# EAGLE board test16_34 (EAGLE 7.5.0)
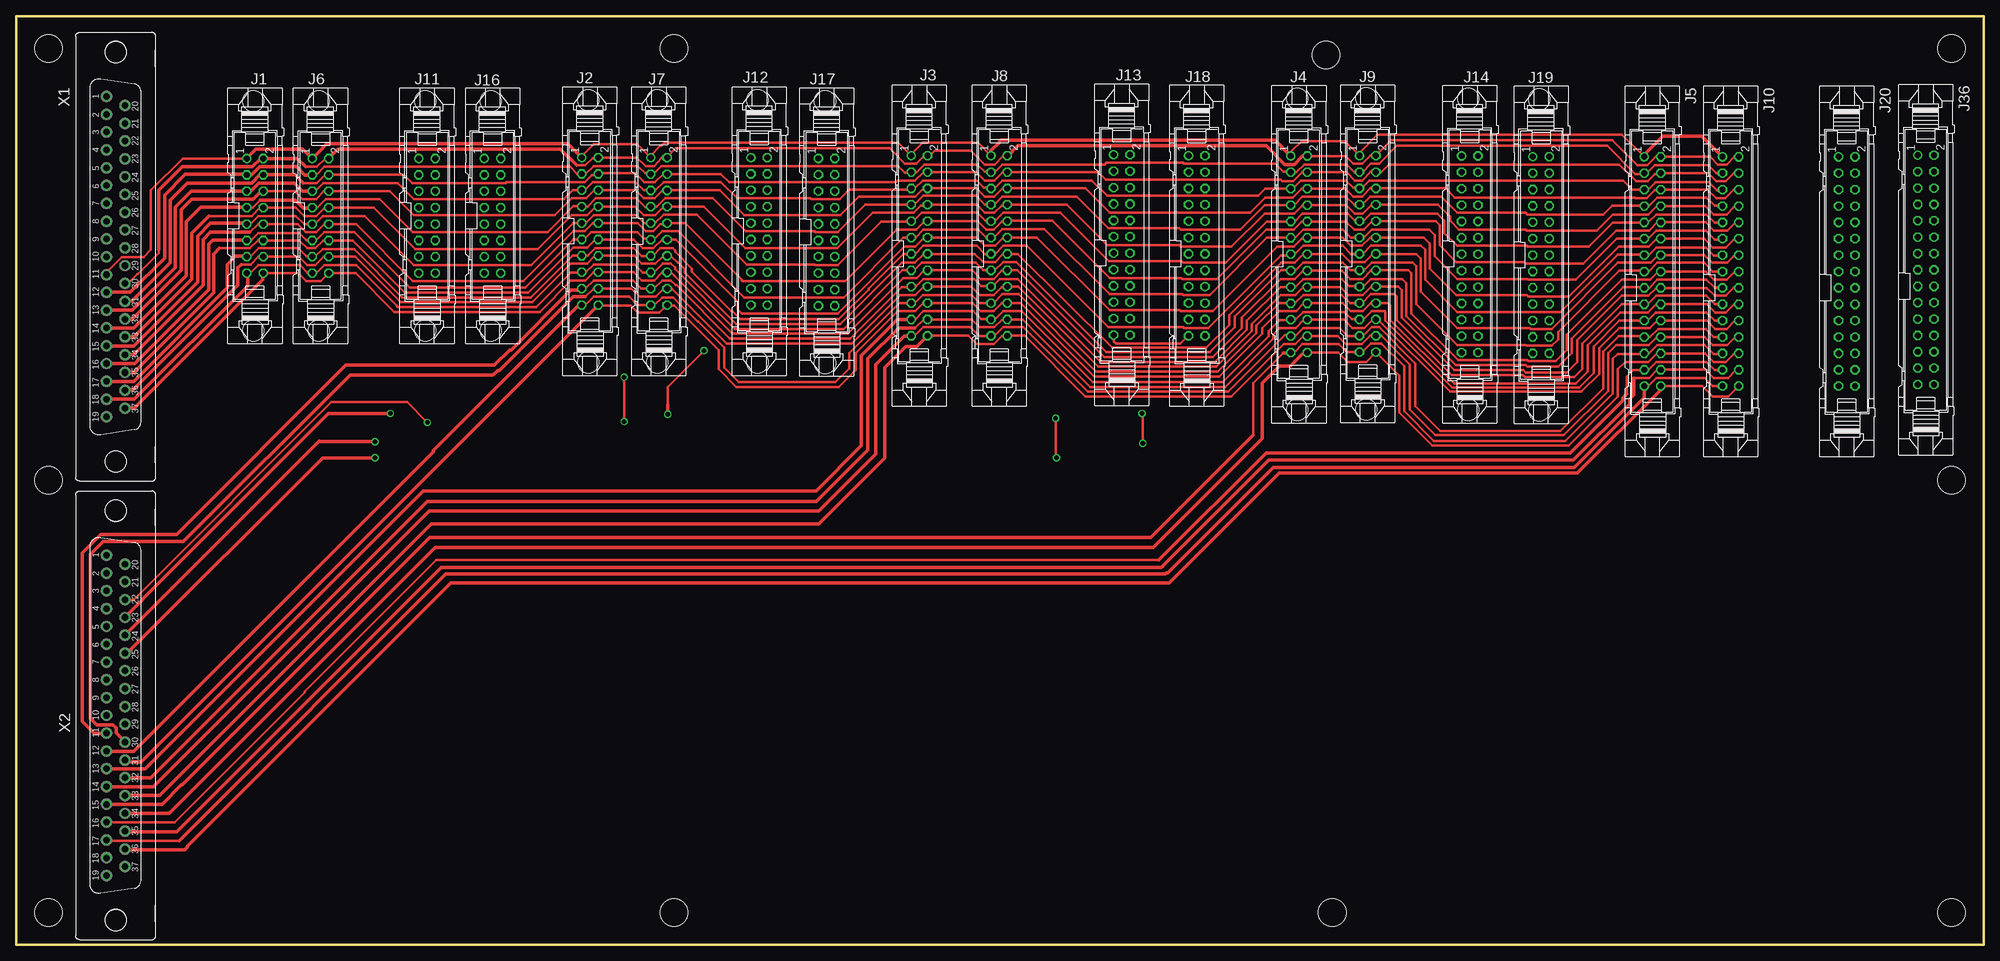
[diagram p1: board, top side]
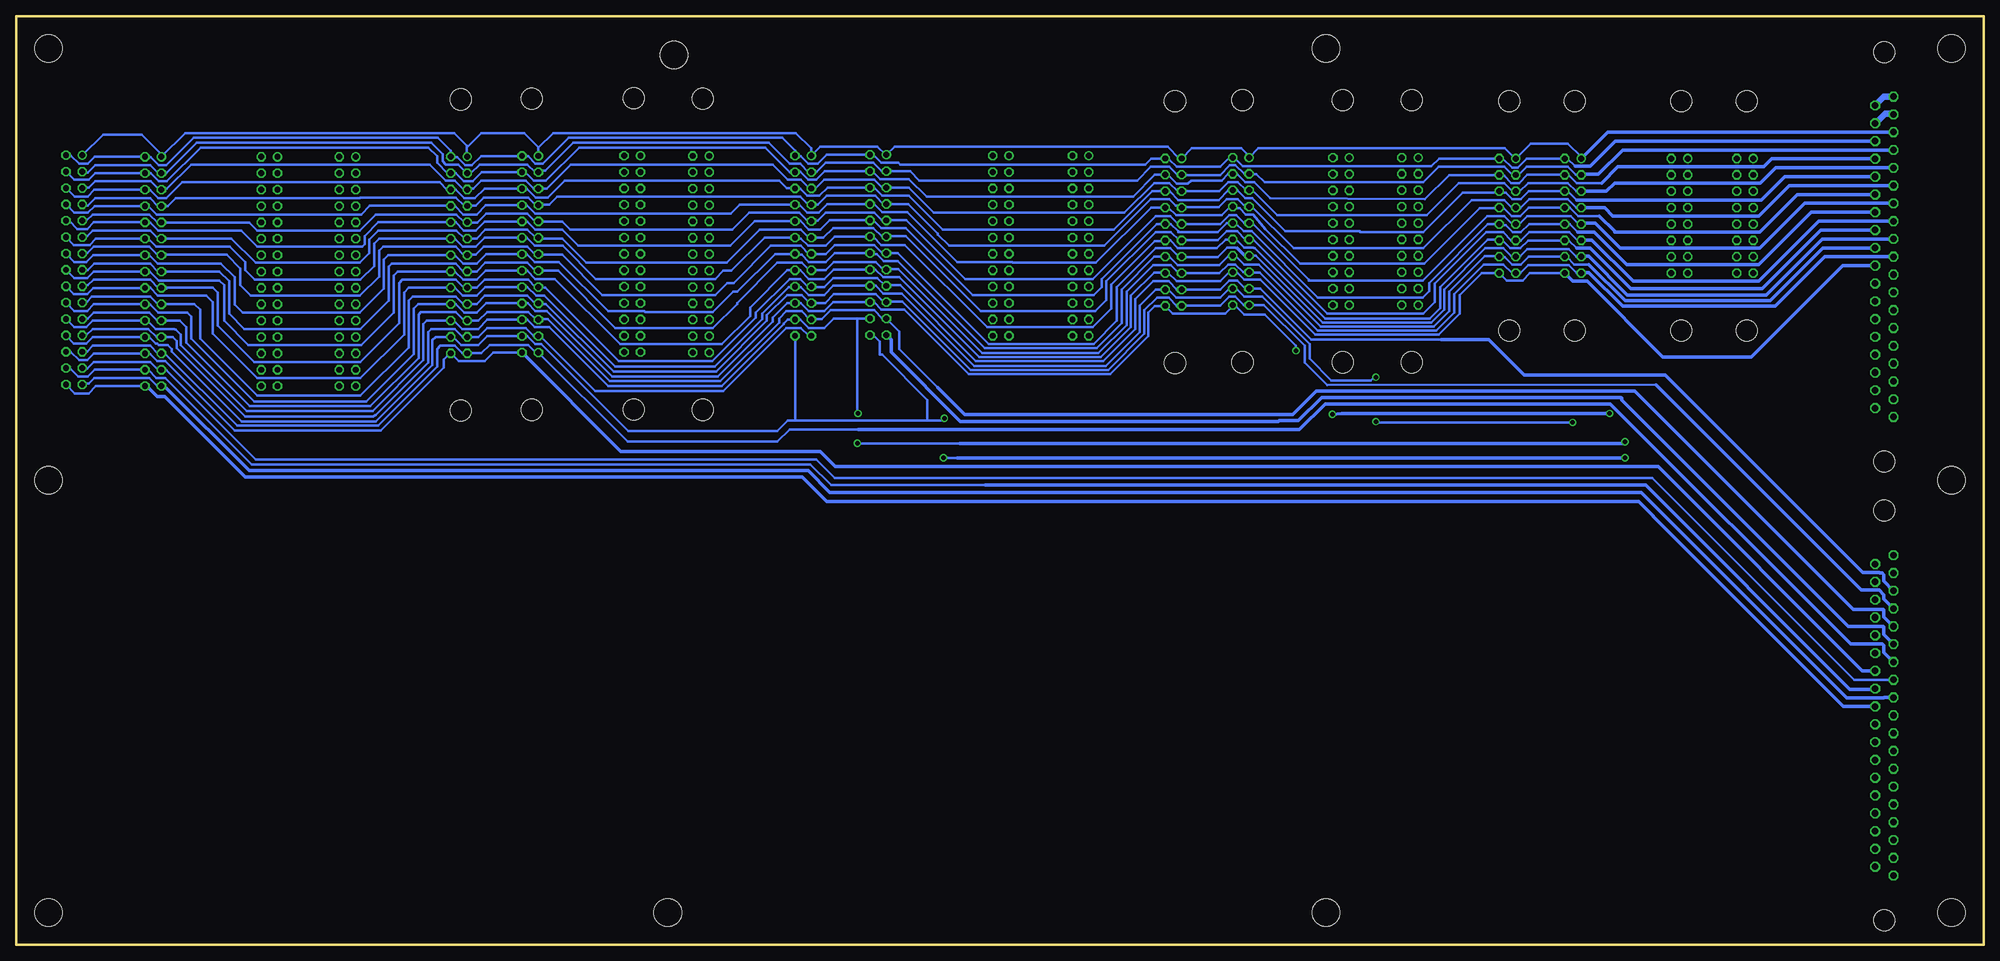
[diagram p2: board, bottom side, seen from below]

Size 305 x 144 mm. Coordinates in mm from the lower left corner, seen from the top.
Outline: 0,144 305,144 305,0 0,0 0,144
Copper layers (1*16): Top 0.035mm / dielectric 1.5mm / Bottom 0.035mm
Design rules "default": minimum track width 10mil, minimum drill 24mil, track to track 8mil, track to pad 8mil, pad to pad 8mil, via to via 8mil, smd to smd 8mil, copper to edge 40mil, drill to drill 8mil, minimum pad ring 10mil, minimum via ring 8mil, stop-mask expansion 4mil, vias tented up to drill 0mil, thermal gap 10mil
Holes 4.3 mm at 5,5 5,139 5,72 300,139 300,72 300,5 102,139 203,138 102,5 204,5

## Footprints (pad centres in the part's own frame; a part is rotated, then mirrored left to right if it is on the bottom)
16V = drill 0.914: 1 -8.89,-1.27 | drill 0.914 octagon: 2 -8.89,1.27; 3 -6.35,-1.27; 4 -6.35,1.27; 5 -3.81,-1.27; 6 -3.81,1.27; 7 -1.27,-1.27; 8 -1.27,1.27; 9 1.27,-1.27; 10 1.27,1.27; 11 3.81,-1.27; 12 3.81,1.27; 13 6.35,-1.27; 14 6.35,1.27; 15 8.89,-1.27; 16 8.89,1.27 | hole 3.302: 17.78,-0.254; -17.78,-0.254
20V = drill 0.914: 1 -11.43,-1.27 | drill 0.914 octagon: 2 -11.43,1.27; 3 -8.89,-1.27; 4 -8.89,1.27; 5 -6.35,-1.27; 6 -6.35,1.27; 7 -3.81,-1.27; 8 -3.81,1.27; 9 -1.27,-1.27; 10 -1.27,1.27; 11 1.27,-1.27; 12 1.27,1.27; 13 3.81,-1.27; 14 3.81,1.27; 15 6.35,-1.27; 16 6.35,1.27; 17 8.89,-1.27; 18 8.89,1.27; 19 11.43,-1.27; 20 11.43,1.27 | hole 3.302: 20.32,-0.254; -20.32,-0.254
24V = drill 0.914: 1 -15.24,-1.27 | drill 0.914 octagon: 2 -15.24,1.27; 3 -12.7,-1.27; 4 -12.7,1.27; 5 -10.16,-1.27; 6 -10.16,1.27; 7 -7.62,-1.27; 8 -7.62,1.27; 9 -5.08,-1.27; 10 -5.08,1.27; 11 -2.54,-1.27; 12 -2.54,1.27; 13 0,-1.27; 14 0,1.27; 15 2.54,-1.27; 16 2.54,1.27; 17 5.08,-1.27; 18 5.08,1.27; 19 7.62,-1.27; 20 7.62,1.27; 21 10.16,-1.27; 22 10.16,1.27; 23 12.7,-1.27; 24 12.7,1.27
26V = drill 0.914: 1 -15.24,-1.27 | drill 0.914 octagon: 2 -15.24,1.27; 3 -12.7,-1.27; 4 -12.7,1.27; 5 -10.16,-1.27; 6 -10.16,1.27; 7 -7.62,-1.27; 8 -7.62,1.27; 9 -5.08,-1.27; 10 -5.08,1.27; 11 -2.54,-1.27; 12 -2.54,1.27; 13 0,-1.27; 14 0,1.27; 15 2.54,-1.27; 16 2.54,1.27; 17 5.08,-1.27; 18 5.08,1.27; 19 7.62,-1.27; 20 7.62,1.27; 21 10.16,-1.27; 22 10.16,1.27; 23 12.7,-1.27; 24 12.7,1.27; 25 15.24,-1.27; 26 15.24,1.27 | hole 3.302: 24.13,-0.254; -24.13,-0.254
30V = drill 0.914: 1 -19.05,-1.27 | drill 0.914 octagon: 2 -19.05,1.27; 3 -16.51,-1.27; 4 -16.51,1.27; 5 -13.97,-1.27; 6 -13.97,1.27; 7 -11.43,-1.27; 8 -11.43,1.27; 9 -8.89,-1.27; 10 -8.89,1.27; 11 -6.35,-1.27; 12 -6.35,1.27; 13 -3.81,-1.27; 14 -3.81,1.27; 15 -1.27,-1.27; 16 -1.27,1.27; 17 1.27,-1.27; 18 1.27,1.27; 19 3.81,-1.27; 20 3.81,1.27; 21 6.35,-1.27; 22 6.35,1.27; 23 8.89,-1.27; 24 8.89,1.27; 25 11.43,-1.27; 26 11.43,1.27; 27 13.97,-1.27; 28 13.97,1.27; 29 16.51,-1.27; 30 16.51,1.27
F37V = drill 1.016 octagon: 1 24.841,1.422; 2 22.073,1.422; 3 19.329,1.422; 4 16.561,1.422; 5 13.792,1.422; 6 11.049,1.422; 7 8.28,1.422; 8 5.512,1.422; 9 2.769,1.422; 10 0,1.422; 11 -2.769,1.422; 12 -5.512,1.422; 13 -8.28,1.422; 14 -11.049,1.422; 15 -13.818,1.422; 16 -16.561,1.422; 17 -19.329,1.422; 18 -22.098,1.422; 19 -24.841,1.422; 20 23.47,-1.422; 21 20.701,-1.422; 22 17.932,-1.422; 23 15.189,-1.422; 24 12.421,-1.422; 25 9.652,-1.422; 26 6.909,-1.422; 27 4.14,-1.422; 28 1.372,-1.422; 29 -1.372,-1.422; 30 -4.14,-1.422; 31 -6.909,-1.422; 32 -9.677,-1.422; 33 -12.421,-1.422; 34 -15.189,-1.422; 35 -17.958,-1.422; 36 -20.701,-1.422; 37 -23.47,-1.422 | hole 3.302: 31.75,0; -31.75,0

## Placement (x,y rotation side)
J1  [16V]  37.02,113.03 270 top
J2  [20V]  88.94,110.64 270 top
J3  24VS  [24V]  140,107.12 270 top
J4  [26V]  198.84,107.08 270 top
J5  30V  [30V]  253.62,103.12 270 top
J6  [16V]  47.18,113.03 270 top
J7  [20V]  99.62,110.62 270 top
J8  24VS  [24V]  152.38,107.12 270 top
J9  [26V]  209.5,107.12 270 top
J10  30V  [30V]  265.75,103.12 270 top
J11  [16V]  63.69,113.03 270 top
J12  [20V]  115.17,110.64 270 top
J13  24VS  [24V]  171.38,107.25 270 top
J14  [26V]  225.31,107.08 270 top
J16  [16V]  73.85,113.03 270 top
J17  [20V]  125.62,110.5 270 top
J18  24VS  [24V]  183,107.12 270 top
J19  [26V]  236.37,106.95 270 top
J20  30V  [30V]  283.75,103.12 270 top
J36  30V  [30V]  296,103.38 270 top
X1  [F37V]  15.43,106.68 90 top
X2  [F37V]  15.43,35.56 90 top

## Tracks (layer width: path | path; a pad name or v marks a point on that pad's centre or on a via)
1
  Bottom 0.406: J11.1 62.42,122.17 64.5,124.25 70.25,124.25 J16.1 72.67,121.92 74.25,123.5 112.47,123.5 J12.1 113.89,122.27 115.12,123.5 122.78,123.5 J17.1 124.68,121.93 126.5,123.75 168.84,123.75 J13.1 170.24,122.49 171.5,123.75 180.34,123.75 J18.1 181.74,123.49 184.12,125.88 221.75,125.88 224.04,123.58 J14.1 224.04,123.67 226.25,125.88 232.88,125.88 235.12,123.62 | J19.1 235.12,122.22 235.12,123.62 | 235.12,123.62 235.12,123.88 237.12,125.88 278.78,125.88 J20.1 282.48,122.61 285.5,125.62 291.53,125.62 J36.1
  Bottom 0.506: X1.3 58.33,126.01 J11.1
2
  Bottom 0.406: 63.38,120.75 64.55,121.92 J11.2 70.83,121.92 72.25,120.5 73.12,120.5 74.55,121.92 J16.2 84.45,121.92 85.62,120.75 114.86,120.75 116.19,122.07 J12.2 116.93,122.07 118.38,120.62 125.12,120.62 126.25,121.75 126.72,121.75 J17.2 129.07,121.93 130,121 168,121 168.25,121.25 170.91,121.25 172.15,122.49 J13.2 179.38,122.49 180.75,121.12 182.25,121.12 183.38,122.25 184.16,122.25 J18.2 | 16.84,124.62 X1.22 | J18.2 184.27,122.52 | J18.2 184.27,123.14 186.25,125.12 219.38,125.12 223.38,121.12 224.5,121.12 225.62,122.25 226.51,122.25 J14.2 232.93,122.32 234.38,120.88 235.38,120.88 236.62,122.12 237.56,122.12 J19.2 237.63,123.14 239.62,125.12 277.5,125.12 281.75,120.88 282.88,120.88 284.12,122.12 284.97,122.12 J20.2 292.82,122.17 293.88,121.12 295.25,121.12 296.5,122.38 297.22,122.38 J36.2
  Bottom 0.506: X1.22 57.14,124.61 61,120.75 63.38,120.75
3
  Bottom 0.406: J11.3 63.26,119.38 64.5,120.62 70.88,120.62 72.12,119.38 J16.3 73.13,119.38 74.38,120.62 84.5,120.62 86.88,118.25 111.5,118.25 112.75,119.5 113.86,119.5 J12.3 114.66,119.53 116,120.88 116.88,120.88 118.38,119.38 124.34,119.38 J17.3 125.02,119.39 126.25,120.62 129.12,120.62 131.25,118.5 165,118.5 166.45,119.95 J13.3 170.82,119.95 172.12,121.25 179.5,121.25 180.88,119.88 181.68,119.88 J18.3 182.2,119.83 183.5,121.12 185.12,121.12 188.38,124.38 218.62,124.38 223,120 223.82,120 J14.3 224.53,119.78 225.75,121 233.12,121 234.5,119.62 235.06,119.62 J19.3 235.16,119.66 236.5,121 238.38,121 238.88,121.5 238.88,122.62 240.62,124.38 277,124.38 281.75,119.62 282.47,119.62 J20.3 283.01,119.64 284.25,120.88 292.75,120.88 293.88,119.75 294.6,119.75 J36.3 | 13.87,123.38 X1.4
  Bottom 0.506: X1.4 56.01,123.24 59.75,119.5 62.3,119.5 J11.3
4
  Bottom 0.406: 59.25,118.12 63.12,118.12 64.38,119.38 J11.4 70.75,119.38 72,118.12 73.25,118.12 74.38,119.25 74.99,119.25 J16.4 82.89,119.38 86.63,115.63 110.62,115.75 113.12,118.25 114.5,118.25 115.78,119.53 J12.4 117.09,119.53 118.12,118.5 122.88,118.5 123.38,118 125.13,118 126.52,119.39 J17.4 128.49,119.39 131.88,116 163.88,116 166.62,118.75 171.07,118.75 172.27,119.95 J13.4 179.68,119.95 181,118.62 182.25,118.62 183.5,119.88 184.22,119.88 J18.4 185.07,119.83 188.88,123.62 217.75,123.62 222.88,118.5 224.81,118.5 226.09,119.78 J14.4 232.84,119.78 234.25,118.38 235.62,118.38 236.88,119.62 237.6,119.62 J19.4 238.16,119.66 239.75,121.25 239.75,122.25 241.12,123.62 276.38,123.62 281.62,118.38 282.88,118.38 284.12,119.62 285.01,119.62 J20.4 286.49,119.64 286.5,119.62 292.75,119.62 293.75,118.62 296.01,118.62 J36.4 | X1.23
  Bottom 0.506: X1.23 32.88,121.87 34.12,120.62 56.75,120.62 59.25,118.12
5
  Bottom 0.406: J11.5 63.22,116.84 64.5,118.12 70.62,118.12 72,116.75 72.49,116.75 J16.5 73.09,116.84 74.38,118.12 81.38,118.12 86.38,113.12 109.5,113.12 113.36,116.99 J12.5 114.36,116.99 115.62,118.25 117.12,118.25 118.5,116.88 124.33,116.88 J17.5 124.97,116.85 126.25,118.12 128.62,118.12 133.25,113.5 162.75,113.5 166.66,117.41 J13.5 170.78,117.41 172,118.62 179.75,118.62 181.12,117.25 181.69,117.25 J18.5 182.03,117.28 183.38,118.62 185.38,118.62 187.75,121 219,121 222.75,117.25 J14.5 224.74,117.24 226,118.5 232.88,118.5 234.12,117.25 234.96,117.25 J19.5 235.62,117.11 237,118.5 238.38,118.5 240.88,121 277.88,121 281.62,117.25 282.32,117.25 J20.5 282.85,117.09 284.12,118.38 292.75,118.38 293.75,117.38 294.7,117.38 J36.5 | 13.98,120.5 X1.5
  Bottom 0.506: X1.5 32.28,120.47 34.62,118.12 57.25,118.12 58.5,116.88 62.38,116.88 J11.5
6
  Bottom 0.406: 63.12,115.5 64.47,116.84 J11.6 70.53,116.84 71.75,115.62 73.12,115.62 74.12,116.62 75,116.62 | 16.83,119.12 X1.24 | J16.6 75.12,116.75 75,116.62 | 75,116.62 80.75,116.62 86.88,110.5 96.62,110.5 96.75,110.62 108.25,110.62 113.38,115.75 114.5,115.75 115.74,116.99 J12.6 117.14,116.99 118.62,115.5 124.88,115.5 126.22,116.85 J17.6 128.9,116.85 134.88,110.88 161.38,110.88 166.62,116.12 170.74,116.12 172.02,117.41 J13.6 179.22,117.41 180.5,116.12 182.38,116.12 183.5,117.25 184.24,117.25 J18.6 185.53,117.28 186.75,118.5 220,118.5 222.62,115.88 224.47,115.88 225.84,117.24 J14.6 232.38,117.24 233.88,115.75 235.52,115.75 236.88,117.11 J19.6 238.24,117.11 239.38,118.25 279.25,118.25 281.75,115.75 283,115.75 284.25,117 284.93,117 J20.6 292.9,117.09 293.88,116 295.93,116 J36.6
  Bottom 0.506: X1.24 30.9,119.1 34.5,115.5 63.12,115.5
7
  Bottom 0.406: J11.7 63.17,114.3 64.5,115.62 70.5,115.62 71.88,114.25 72.53,114.25 J16.7 73.17,114.3 74.38,115.5 79.38,115.5 86.88,108 107,108 113.45,114.45 J12.7 114.45,114.45 115.62,115.62 117.38,115.62 118.62,114.38 124.29,114.38 J17.7 124.67,114.62 125.25,114.62 126.25,115.62 129.12,115.62 136.38,108.38 160.38,108.38 162.12,110.12 162.12,110.25 166.75,114.87 J13.7 170.62,114.87 171.88,116.12 179.38,116.12 180.75,114.75 J18.7 182.25,114.75 183.5,116 221.12,116 222.38,114.75 224,114.75 J14.7 224.45,114.7 225.62,115.88 232.5,115.88 233.75,114.62 235.04,114.62 J19.7 235.57,114.58 236.88,115.88 251.62,115.88 251.75,115.75 280.25,115.75 281.5,114.5 282.43,114.5 J20.7 283.06,114.56 284.25,115.75 292.75,115.75 293.88,114.62 294.55,114.62 J36.7 | 13.9,117.62 X1.6
  Bottom 0.506: X1.6 30.15,117.73 34.88,113 57.5,113 58.8,114.3 J11.7
8
  Bottom 0.406: 59.62,113 62.88,113 64.17,114.3 J11.8 70.58,114.3 71.88,113 73.19,113 74.5,114.3 J16.8 75.17,114.25 78.12,114.25 86.75,105.62 106,105.62 111.38,111 113.25,113.25 114.38,113.25 115.38,114.25 116.37,114.25 116.44,114.19 J12.8 116.8,114.45 118.12,113.12 125.21,113.12 126.39,114.31 J17.8 129.06,114.31 137.62,105.75 150.5,105.75 150.62,105.88 159.12,105.88 166.88,113.62 170.75,113.62 172,114.87 J13.8 179.25,114.87 180.62,113.5 182.4,113.5 183.65,114.75 J18.8 192.88,114.75 194.25,113.38 224.51,113.38 225.84,114.7 J14.8 232.18,114.7 233.62,113.25 235.69,113.25 237.01,114.58 J19.8 250.18,114.58 251.5,113.25 283.21,113.25 284.52,114.56 J20.8 292.82,114.56 293.88,113.5 295.96,113.5 J36.8 | 17.29,116.25 17.38,116.33
  Bottom 0.506: X1.25 17.38,116.33 28.92,116.33 34.75,110.5 57.25,110.5 57.25,110.62 59.62,113
9
  Bottom 0.406: J11.9 62.76,111.76 64,113 70.75,113 72,111.75 J16.9 73.14,111.76 74.38,113 77,113 87,103 104.61,103 104.61,103.11 113.25,111.75 113.73,111.75 J12.9 113.93,111.88 114.62,111.88 115.88,113.12 117,113.12 118.36,111.77 J17.9 124.89,111.77 126.12,113 128.38,113 138.12,103.25 157.88,103.25 167,112.38 170.06,112.38 J13.9 170.83,112.33 172,113.5 179.5,113.5 180.75,112.25 181.69,112.25 J18.9 182.33,112.2 183.62,113.5 191.38,113.5 194,110.88 219.12,110.88 220.38,112.12 224.01,112.12 J14.9 224.53,112.16 225.75,113.38 232.12,113.38 233.5,112 235.06,112 J19.9 235.53,112.03 236.75,113.25 249.25,113.25 251.75,110.75 267.62,110.75 268.88,112 282.46,112 J20.9 283.14,112.02 284.38,113.25 293.12,113.25 294.12,112.25 294.71,112.25 J36.9 | 13.97,115 X1.7
  Bottom 0.506: X1.7 27.79,114.96 34.75,108 56.38,108 60.25,111.88 62.3,111.88 J11.9
10
  Bottom 0.406: 16.82,113.62 X1.26 | 62.95,110.5 64.21,111.76 J11.10 70.49,111.76 71.75,110.5 73,110.5 74.12,111.62 74.98,111.62 J16.10 76.86,111.76 86,102.62 86,101.38 87,100.38 103.25,100.38 113.5,110.62 114.75,110.62 116.03,111.91 J12.10 117.34,111.91 118.75,110.5 124.88,110.5 124.88,110.62 126,111.75 126.88,111.75 J17.10 128.23,111.77 136.75,103.25 136.75,102 138,100.75 156.75,100.75 167.12,111.12 170.94,111.12 172.15,112.33 J13.10 178.92,112.33 180.38,110.88 182.12,110.88 183.5,112.25 184.22,112.25 J18.10 190.5,112.2 194.33,108.38 217.88,108.38 220.38,110.88 224.5,110.88 225.75,112.12 226.55,112.12 J14.10 232.34,112.16 233.75,110.75 235.6,110.75 236.88,112.03 J19.10 248.84,112.03 251,109.88 251,108.62 251.38,108.25 267.62,108.25 270.12,110.75 283,110.75 284.25,112 285,112 J20.10 292.99,112.02 294,111 295.5,111 296.75,112.25 297.25,112.25 J36.10
  Bottom 0.506: X1.26 26.79,113.59 34.88,105.5 55.38,105.5 60.38,110.5 62.95,110.5
11
  Bottom 0.406: 13.95,112.25 X1.8 | J11.11 62.97,109.22 64.25,110.5 70.5,110.5 71.78,109.22 J16.11 73.22,109.22 74.5,110.5 77.12,110.5 85.12,102.5 85.12,99.62 86.88,97.88 101.75,97.88 113.25,109.38 J12.11 114.5,109.37 115.75,110.62 117.38,110.62 118.77,109.23 J17.11 124.73,109.23 126,110.5 128.38,110.5 136,102.88 136,100 137.75,98.25 155.5,98.25 167.12,109.88 170.02,109.88 J13.11 170.79,109.79 172.12,111.12 178.38,111.12 179.88,109.62 181.69,109.62 J18.11 182.16,109.67 183.38,110.88 189.75,110.88 194.88,105.75 216.62,105.75 220.38,109.5 223.93,109.5 J14.11 224.5,109.62 225.75,110.88 232.25,110.88 233.62,109.5 J19.11 235.5,109.5 236.75,110.75 248.88,110.75 250.25,109.38 250.25,107.25 251.75,105.75 267.88,105.75 271.62,109.5 282.45,109.5 J20.11 282.98,109.47 284.25,110.75 293.12,110.75 294,109.88 294.58,109.88 J36.11
  Bottom 0.506: X1.8 25.56,112.19 34.88,102.88 54.38,102.88 60.75,109.25 62.39,109.25 J11.11
12
  Bottom 0.406: 63.12,108 64.34,109.22 J11.12 70.66,109.22 71.88,108 73.38,108 74.62,109.25 75.09,109.25 J16.12 75.28,109.38 76.88,109.38 84.25,102 84.25,98.75 85.88,97.12 102.12,97.12 113,108 113.12,108 113.25,108.12 114.62,108.12 115.87,109.37 J12.12 117.5,109.37 118.88,108 124.92,108 126.14,109.23 J17.12 127,109.12 128.5,109.12 135.25,102.38 135.25,98.62 138.12,95.75 154.5,95.75 167.25,108.5 170.88,108.5 172.16,109.79 J13.12 178.09,109.79 179.5,108.38 182.25,108.38 183.38,109.5 184.1,109.5 J18.12 189,109.67 194.16,104.5 195.38,104.5 196.62,103.25 215.12,103.25 220.25,108.38 224.59,108.38 225.84,109.62 J14.12 232.38,109.62 233.75,108.25 235.76,108.25 237.01,109.5 J19.12 248.75,109.5 249.5,108.75 249.5,105.25 251.62,103.12 268,103.12 269.5,104.62 269.5,105.88 271.88,108.25 283.3,108.25 284.52,109.47 J20.12 292.65,109.47 293.62,108.5 296.05,108.5 J36.12 | 16.8,110.88 X1.27
  Bottom 0.506: X1.27 25.3,110.82 34.38,101.75 54.75,101.75 61,108 63.12,108
13
  Bottom 0.406: J11.13 63.18,106.68 64.38,107.88 70.75,107.88 71.88,106.75 72.51,106.75 J16.13 72.65,106.75 73.25,106.75 74.5,108 77.25,108 83.62,101.62 83.62,98.5 85.62,96.5 102.5,96.5 112.83,106.83 J12.13 | 13.96,109.5 X1.9 | 115.75,108 115.88,108 116,108.12 117.25,108.12 118.75,106.62 124.29,106.62 J17.13 124.81,106.69 126.12,108 128.38,108 134.38,102 134.38,96.75 138,93.12 154.25,93.12 168.38,107.25 J13.13 170.75,107.25 172,108.5 178.12,108.5 179.5,107.12 J18.13 182.12,107.12 183.38,108.38 188,108.38 193.75,102.62 194.75,102.62 196.62,100.75 214.12,100.75 220.38,107 223.97,107 J14.13 | 223.84,106.88 J14.13 | J14.13 224.58,107.08 225.75,108.25 232.5,108.25 233.75,107 235.05,107 J19.13 235.58,106.95 236.88,108.25 248.12,108.25 248.75,107.62 248.75,103.62 251.75,100.62 268.62,100.62 270.25,102.25 270.25,104.88 272.38,107 282.42,107 J20.13 283.06,106.94 284.38,108.25 293,108.25 294,107.25 294.67,107.25 J36.13
  Bottom 0.506: X1.9 25.05,109.45 33.75,100.75 55.25,100.75 61.25,106.75 62.35,106.75 J11.13 | J12.13 114.58,106.83 115.75,108
14
  Bottom 0.406: 61.25,105.5 63.5,105.5 64.68,106.68 J11.14 70.57,106.68 71.75,105.5 73.12,105.5 74.25,106.62 75.06,106.62 J16.14 75.19,106.75 77.38,106.75 82.88,101.25 82.88,98.25 85.25,95.88 102.75,95.88 112.38,105.5 114.62,105.5 115.94,106.81 116.44,106.81 J12.14 117.05,106.83 118.5,105.38 124.95,105.38 126.27,106.69 J17.14 128.56,106.69 133.62,101.62 133.62,96.38 137.5,92.5 154.88,92.5 168.38,106 170.5,106 171.62,107.12 172.52,107.12 J13.14 178.12,107.25 179.5,105.88 182.12,105.88 183.25,107 184.15,107 J18.14 187.38,107.12 193.25,101.25 193.88,101.25 197,98.12 207.5,98.12 207.62,98.25 213.25,98.25 220.88,105.88 224.63,105.88 225.84,107.08 J14.14 232.17,107.08 233.62,105.62 235.68,105.62 237.01,106.95 J19.14 247.29,106.95 248,106.25 248,101.75 251.75,98 269.88,98 271.12,99.25 271.12,103.5 273.25,105.62 283.08,105.62 284.39,106.94 J20.14 293.06,106.94 294.12,105.88 295.96,105.88 J36.14 | 16.78,108.12 X1.28
  Bottom 0.506: X1.28 24.95,108.05 33.12,99.88 55.62,99.88 61.25,105.5
15
  Bottom 0.406: J11.15 63.14,104.14 64.38,105.38 70.62,105.38 71.88,104.12 72.56,104.12 J16.15 73.14,104.14 74.5,105.5 77.5,105.5 82.12,100.88 82.12,98 84.88,95.25 103.25,95.25 112.25,104.25 113.86,104.25 J12.15 114.79,104.29 116,105.5 117.12,105.5 118.5,104.12 124.33,104.12 J17.15 124.78,104.15 126,105.38 128.75,105.38 132.88,101.25 132.88,96.12 137.25,91.75 155.25,91.75 168.25,104.75 170.06,104.75 J13.15 170.59,104.71 171.75,105.88 178.25,105.88 179.5,104.62 181.69,104.62 J18.15 182.09,104.58 183.25,105.75 187,105.75 193.25,99.5 193.25,99.38 197,95.62 212.12,95.62 221,104.5 224,104.5 J14.15 224.54,104.54 225.75,105.75 232.25,105.75 233.62,104.38 235.06,104.38 J19.15 235.66,104.42 236.88,105.62 246.75,105.62 247.25,105.12 247.25,99.88 251.62,95.5 269.62,95.5 272,97.88 272,102.88 273.5,104.38 282.46,104.38 J20.15 283.02,104.39 284.25,105.62 292.88,105.62 293.88,104.62 294.71,104.62 J36.15 | 13.95,106.62 X1.10
  Bottom 0.506: X1.10 24.7,106.68 32.38,99 56,99 61.25,104.25 62.31,104.25 J11.15
16
  Bottom 0.406: J11.16 70.36,104.14 71.5,103 73.98,103 J16.16 77.86,104.14 81.25,100.75 81.25,97.88 84.5,94.62 103.62,94.62 112.12,103.12 114.62,103.12 115.79,104.29 J12.16 116.96,104.29 118.38,102.88 125.12,102.88 126.39,104.15 J17.16 127,104.25 128.62,104.25 132.25,100.62 132.25,95.75 136.88,91.12 155.75,91.12 168.12,103.5 170.62,103.5 171.84,104.71 J13.16 178.29,104.71 179.75,103.25 182.12,103.25 183.5,104.62 184.23,104.62 J18.16 185.5,104.58 191.25,98.83 191.25,97.5 195.62,93.12 211.38,93.12 221.5,103.25 224.5,103.25 225.75,104.5 226.54,104.5 J14.16 232.21,104.54 233.62,103.12 235.72,103.12 237.01,104.42 J19.16 245.84,104.42 246.5,103.75 246.5,98 251.5,93 269,93 272.75,96.75 272.75,102.25 273.5,103 282.88,103 284.27,104.39 J20.16 292.98,104.39 294,103.38 296,103.38 J36.16 | 16.79,105.25 X1.29
  Bottom 0.506: X1.29 21.88,105.31 36.06,91.12 49.75,91.12 61.5,102.88 63.7,102.88 J11.16
17
  Bottom 0.406: 84.12,93.88 104.25,93.88 112.12,101.75 J12.17 114.5,101.75 115.75,103 117,103 118.38,101.62 124.34,101.62 J17.17 125.11,101.61 126.38,102.88 128.75,102.88 131.5,100.12 131.5,95.5 136.5,90.5 156.25,90.5 168,102.25 170.03,102.25 J13.17 170.29,102.17 171.5,103.38 178.38,103.38 179.75,102 181.69,102 J18.17 182.29,102.05 183.5,103.25 185.12,103.25 190.38,98 190.38,97.25 197.12,90.5 211.62,90.5 223,101.88 223.92,101.88 J14.17 224.5,102 225.62,103.12 232.38,103.12 233.62,101.88 J19.17 235.62,101.88 236.88,103.12 245.12,103.12 245.62,102.62 245.62,96.38 251.62,90.38 268.12,90.38 273.75,96 273.75,101.12 274.5,101.88 281.62,101.88 281.75,101.75 282.38,101.75 J20.17 282.98,101.86 284.25,103.12 293,103.12 293.88,102.25 294.58,102.25 J36.17
  Bottom 0.506: X2.3 15.5,56.38 15.5,57.38 15.75,57.62 16.12,57.62 16.25,57.75 18.75,57.75 49.38,88.38 71.25,88.38 76.75,93.88 84.12,93.88
18  (via drill 0.7)
  Top 0.406: X2.22 18.24,53.49 48.88,84.12 60.62,84.12 v63.75,81 | v94.25,81.12 v94.25,88
  Bottom 0.406: v63.75,81 94.12,81 v94.25,81.12 | 116.44,101.69 115.81,101.69 114.62,100.5 111.88,100.5 104.5,93.12 104.5,90.88 101.12,87.5 95,87.5 94.5,88 v94.25,88 | 116.44,101.69 117.06,101.69 118.38,100.38 125.16,100.38 126.39,101.61 J17.18 126.91,101.62 128.38,101.62 130.88,99.12 130.88,95 136.12,89.75 156.5,89.75 167.75,101 170.62,101 171.79,102.17 J13.18 178.33,102.17 179.75,100.75 182.12,100.75 183.38,102 184.22,102 J18.18 184.31,102 185.25,102 189.38,97.88 189.38,97 196.75,89.62 212.12,89.62 223.12,100.62 224.38,100.62 225.75,102 J14.18 232.25,102 233.62,100.62 235.76,100.62 237.01,101.88 J19.18 244.12,101.88 244.88,101.12 244.88,94.62 251.62,87.88 267.62,87.88 274.5,94.75 274.5,99.62 275.5,100.62 283.04,100.62 283.04,100.67 284.25,101.88 285,101.88 J20.18 293.02,101.86 294,100.88 296.04,100.88 J36.18
  Bottom 0.506: 116.44,101.69 J12.18
19
  Bottom 0.406: 50.81,86.81 50.88,86.88 101.75,86.75 105.25,90.25 105.25,92.88 111.58,99.21 J12.19 114.71,99.21 116,100.5 117,100.5 118.38,99.12 124.3,99.12 J17.19 125.07,99.07 126.38,100.38 128.12,100.38 130.12,98.38 130.12,94.75 135.75,89.12 157,89.12 167.62,99.75 169.99,99.75 J13.19 170.5,99.63 171.75,100.88 178.25,100.88 179.62,99.5 J18.19 182,99.5 183.25,100.75 185.5,100.75 188.62,97.62 188.62,96.75 196.5,88.88 212.38,88.88 222.88,99.38 223.96,99.38 J14.19 | 224,99.5 J14.19 | J14.19 224.59,99.46 225.75,100.62 232.38,100.62 233.62,99.38 235.06,99.38 J19.19 235.71,99.33 236.88,100.5 243.5,100.5 244.12,99.88 244.12,92.62 251.62,85.12 267.62,85.12 276.5,94 276.5,98.5 277.38,99.38 282.42,99.38 J20.19 283.06,99.31 284.25,100.5 293.25,100.5 294,99.75 294.55,99.75 J36.19
  Bottom 0.506: X2.4 15.5,53.61 15.5,54.25 16.25,55 19,55 50.81,86.81
20  (via drill 0.7)
  Top 0.406: 101,83.78 101,86.5 v106.62,92.12
  Top 0.506: X2.23 19.62,53.52 19.62,53.62 48.38,82.38 v58,82.38 | v101,82.25 101,83.78
  Bottom 0.406: v106.62,92.12 106.62,92.88 111.5,97.75 114.62,97.75 116.08,99.21 J12.20 116.44,99.06 117.62,97.88 125.7,97.88 J17.20 126.97,99 128.5,99 129.5,98 129.5,94.38 135.38,88.5 157.38,88.5 167.38,98.5 170.88,98.5 172,99.63 J13.20 178.37,99.63 179.75,98.25 182.12,98.25 183.38,99.5 J18.20 185.5,99.5 187.75,97.25 187.75,96.62 196.25,88.12 212.62,88.12 222.75,98.25 224.5,98.25 225.71,99.46 J14.20 232.16,99.46 233.62,98 235.55,98 236.88,99.33 J19.20 242.66,99.33 243.38,98.62 243.38,91.62 250.75,84.25 268.12,84.25 277.88,94 277.88,97.38 278.5,98 283,98 284.25,99.25 284.95,99.25 J20.20 292.94,99.31 294,98.25 295.95,98.25 J36.20
  Bottom 0.506: v58,82.38 99.5,82.38 v101,82.25
21
  Bottom 0.406: 162.12,86.38 168.12,92.38 168.12,95.11 J13.21 170.72,97.09 172,98.38 178.75,98.38 180.12,97 181.69,97 J18.21 181.97,96.97 183.25,98.25 185.62,98.25 186.75,97.12 186.75,96.5 195.88,87.38 213,87.38 222.62,97 223.97,97 J14.21 224.42,96.92 225.62,98.12 232,98.12 233.38,96.75 235.05,96.75 J19.21 235.54,96.8 236.88,98.12 242.25,98.12 242.62,97.75 242.62,91 250.12,83.5 268.75,83.5 278.62,93.38 278.62,95.75 279.62,96.75 282.45,96.75 J20.21 283.15,96.78 284.38,98 293,98 293.88,97.12 294.63,97.12 J36.21
  Bottom 0.506: X2.5 15.5,50.84 15.5,51.88 15.62,52 20.25,52 54.12,85.88 103.5,85.88 107.12,82.25 158,82.25 162.12,86.38
22  (via drill 0.7)
  Top 0.406: v174.62,77.75 174.62,82.25 v174.5,82.38
  Top 0.506: X2.24 46.87,78 | 46.87,78 47,78.12 | v55.62,78 46.87,78
  Bottom 0.406: 172.78,97.09 J13.22 172.68,97.12 174.5,97.12 | 174.62,82.75 174.62,97 174.5,97.12 | 174.62,82.75 174.62,82.5 v174.5,82.38 | v174.5,82.38 174.38,82.25 | 158.75,77.75 v174.62,77.75 | v174.5,82.38 174.5,82.62 174.62,82.75 | 174.5,97.12 178.25,97.12 179.75,95.62 182.12,95.62 183.47,96.97 J18.22 185.38,96.97 186,96.34 186,96.25 195.62,86.62 213.25,86.62 222.38,95.75 224.62,95.75 225.79,96.92 J14.22 231.96,96.92 233.38,95.5 235.84,95.5 237.13,96.8 J19.22 241.33,96.8 241.88,96.25 241.88,90.62 249.75,82.75 269.25,82.75 279.5,93 279.5,94.62 280.25,95.38 280.38,95.38 280.5,95.5 283.38,95.5 284.65,96.78 J20.22 293.1,96.78 294.12,95.75 296,95.75 J36.22
  Bottom 0.506: 158.75,77.75 55.88,77.75 v55.62,78
23
  Top 0.406: J18.23 180.43,93.25 170.5,93.25 170.1,93.52 J13.23
  Bottom 0.406: J18.23 182.18,94.42 183.38,95.62 185.62,95.62 195.38,85.88 215.25,85.88 223.5,94.12 223.79,94.12 J14.23 224.75,94.38 226,95.62 232,95.62 233.38,94.25 J19.23 235.75,94.25 237,95.5 240.62,95.5 241.12,95 241.12,90.25 249.25,82.12 249.38,82.12 249.62,81.88 269.5,81.88 280.12,92.5 280.12,93.62 280.75,94.25 282.46,94.25 J20.23 283.24,94.23 284.5,95.5 293.12,95.5 294.12,94.5 294.71,94.5 J36.23
  Bottom 0.506: X2.6 15.5,48.1 15.5,49.25 15.62,49.38 21,49.38 56.12,84.5 56.12,84.75 56.25,84.88 102.62,84.88 106.25,81.25 109.25,81.25 109.38,81.12 158.62,81.12 169.38,91.88 169.38,93.82 J13.23
24  (via drill 0.7)
  Top 0.406: v161.12,81.62 161.12,75.62 v161.25,75.5
  Top 0.506: v55.62,75.5 47.5,75.5 17.38,45.38 17.02,45.38 X2.25
  Bottom 0.406: v161.25,75.5 159.12,75.5 | J18.24 184.27,81.48 184.5,81.25 | 184.5,81.25 163.88,81.25 | 163.88,81.25 161.5,81.25 v161.12,81.62 | 163.88,81.25 163.75,81.38 163.75,84.5 170.75,91.5 171.12,91.5 171.12,93.5 172.15,94.52 172.62,94.52 J13.24 | 184.5,81.25 185.38,81.25 187,79.62 210.12,79.62 223.62,93.12 224.5,93.12 225.75,94.38 225.88,94.38 J14.24 232,94.38 233.38,93 236,93 237.26,94.25 J19.24 240,94.25 240.5,93.75 240.5,89.88 249.25,81.12 270,81.12 280.88,92 280.88,92.38 281.5,93 282.91,93 283.16,93.25 283.38,93.25 284.36,94.23 J20.24 293.14,94.23 294.12,93.25 296.04,93.25 J36.24
  Bottom 0.506: 159.12,75.5 v55.62,75.5
25
  Bottom 0.406: 174.5,79.88 185.12,79.88 187,78 210.21,78 J14.25 224.47,91.84 225.62,93 231.62,93 232.88,91.75 235.06,91.75 J19.25 235.84,91.72 237,92.88 239.25,92.88 239.75,92.38 239.75,89.62 248.88,80.5 270.75,80.5 281.88,91.62 282.41,91.62 J20.25 283.07,91.69 284.25,92.88 293.12,92.88 294,92 294.68,92 J36.25
  Bottom 0.506: X2.7 15.5,45.33 15.5,46.38 15.75,46.62 20.62,46.62 57.88,83.88 102.12,83.88 106.12,79.88 174.5,79.88
26
  Bottom 0.406: J14.26 231.03,91.84 232.38,90.5 236.42,90.5 J19.26 237.78,91.72 238.75,90.75 238.75,89.5 248.5,79.75 271.12,79.75 281.88,90.5 283.12,90.5 284.25,91.62 284.95,91.62 J20.26 292.93,91.69 294,90.62 295.25,90.62 296.5,91.88 297.2,91.88 J36.26
  Bottom 0.506: X2.26 18.84,42.47 50.5,74.12 178,74.12 180.38,76.5 211.25,76.5 J14.26
27
  Bottom 0.406: X2.8 20.07,41.07 51.38,72.38 178.12,72.38 181,75.25 267.88,75.25 281.62,89 282.32,89 J20.27 283.03,89.16 284.25,90.38 293,90.38 294,89.38 294.7,89.38 J36.27
28
  Bottom 0.406: 154.75,71.25 178.62,71.25 181.88,74.5 268.5,74.5 281.88,87.88 283.25,87.88 284.53,89.16 J20.28 292.85,89.16 293.88,88.12 295.38,88.12 296.62,89.38 297.24,89.38 J36.28
  Bottom 0.506: 154.75,71.25 52.38,71.25 20.75,39.62 16.93,39.62 X2.27
29
  Bottom 0.406: J20.29 283.12,86.61 284.38,87.88 292.88,87.88 293.75,87 294.6,87 J36.29
  Bottom 0.506: X2.9 15.42,38.33 15.5,38.25 21.25,38.25 53.12,70.12 178.88,70.12 182.25,73.5 268.88,73.5 281.88,86.5 282.37,86.5 J20.29
30
  Bottom 0.406: J20.30 292.63,86.61 293.75,85.5 295.9,85.5 J36.30
  Bottom 0.506: J20.30 284.74,86.61 283.12,85 282,85 269.5,72.5 183.12,72.5 179.38,68.75 53.5,68.75 51.25,66.5 51.25,66.38 21.81,36.93 X2.28
+5V
  Bottom 1.016: X1.21 16.74,127.38 15.25,128.88 14.13,128.88 X1.2
GND
  Bottom 1.016: X1.1 15.48,131.52 X1.20
L1
  Top 0.406: J2.1 87.67,122.3 89.5,124.12 96.28,124.12 J7.1 98.36,122.36 99.88,123.88 100,123.88 100.5,124.38 136.72,124.38 J3.1 138.73,122.61 140.5,124.38 149.09,124.38 J8.1 | J1.1 25.8,121.92 20.88,117 20.88,107.75 19.75,106.62 16.38,106.62 14.38,104.62 14.38,104.28 X1.11 | J4.1 197.57,122.94 199.25,124.62 205.97,124.62 J9.1 208.23,122.86 211,125.62 248.91,125.62 J5.1
  Top 0.506: J1.1 35.75,122 37.12,123.38 44.45,123.38 J6.1 47.5,123.5 47.5,123.62 48.12,124.25 85.49,124.25 J2.1 | J8.1 151.1,123.11 152.38,124.38 152.38,124.5 152.62,124.75 195.14,124.75 J4.1 | J5.1 252.35,122.48 255.25,125.38 261.28,125.38 J10.1
L2
  Top 0.406: 86.88,120.88 88.25,120.88 89.38,122 90.14,122 J2.2 96.18,122.07 97.62,120.75 98.88,120.75 100.06,122.06 J7.2 100.89,122.14 102.25,123.5 135.38,123.5 137.75,121.12 139.53,121.12 140.77,122.36 J3.2 141.62,122.36 142.38,123.12 148,123.12 150.12,121 151.66,121 153.02,122.36 J8.2 | J6.2 47.92,121.92 46.62,120.62 44.88,120.62 | 22.12,107.75 22.12,107.25 18.88,104 18.75,104 17.38,102.62 16.94,102.62 X1.30 | J4.2 202.68,122.32 202.75,122.25 206.12,122.25 207.25,121.12 208.62,121.12 209.88,122.38 210.76,122.38 J9.2 210.77,122.39 213.12,124.75 247.38,124.75 251.25,120.88 252.84,120.88 254.15,122.17 J5.2 262.57,122.17 263.75,121 265.12,121 266.3,122.17 J10.2
  Top 0.506: 22.12,107.75 22.12,117 25.75,120.62 36.62,120.62 37.92,121.92 J1.2 43.58,121.92 44.88,120.62 | J6.2 48.45,121.95 49.88,123.38 84.38,123.38 86.88,120.88 | J8.2 153.74,122.36 155.25,123.88 193.75,123.88 196.62,121 198.12,121 199.38,122.25 200.04,122.25 J4.2
L3
  Top 0.406: J6.3 46.5,119.38 47.75,120.62 85.88,120.62 87,119.5 87.64,119.5 J2.3 88.28,119.53 89.5,120.75 96.38,120.75 97.5,119.62 98.25,119.62 J7.3 98.77,119.52 100,120.75 136.75,120.75 137.75,119.75 138.66,119.75 J3.3 139.57,119.83 140.75,121 149,121 150.12,119.88 151.06,119.88 J8.3 151.7,119.83 152.88,121 168.75,121 169,121.25 180.88,121.25 181,121.12 195.12,121.12 196.38,119.88 197.47,119.88 J4.3 198.41,119.78 199.62,121 206.25,121 207.5,119.75 208.16,119.75 J9.3 208.7,119.83 210,121.12 211.25,121.12 214,123.88 246.62,123.88 251,119.5 252.22,119.5 J5.3 252.76,119.64 254,120.88 262.25,120.88 263.5,119.62 264.47,119.62 J10.3
  Top 0.506: X1.12 17.67,101.17 23,106.5 23,116.25 26.25,119.5 35.63,119.5 J1.3 36.51,119.38 37.75,120.62 43.5,120.62 44.75,119.38 J6.3
L4
  Top 0.406: 44.5,118.12 46.62,118.12 47.88,119.38 J6.4 60.12,119.38 61.38,118.12 75.88,118.12 76,118.25 88.12,118.25 89.25,119.38 90.06,119.38 J2.4 90.31,119.62 96,119.62 97.38,118.25 99,118.25 100.27,119.52 J7.4 109.23,119.52 110.5,118.25 136.38,118.25 136.62,118.5 139.32,118.5 140.65,119.83 J3.4 148.8,119.83 150.12,118.5 151.62,118.5 152.88,119.75 153.57,119.75 J8.4 167.68,119.83 168.88,118.62 196,118.62 196.25,118.38 197.96,118.38 199.36,119.78 J4.4 206.22,119.78 207.5,118.5 208.62,118.5 210,119.88 210.72,119.88 J9.4 211.57,119.83 212.75,121 248.5,121 251.12,118.38 252.88,118.38 254,119.5 254.76,119.5 J5.4 262.24,119.64 263.5,118.38 265,118.38 266.25,119.62 267.01,119.62 J10.4
  Top 0.506: X1.31 17.9,99.77 23.88,105.75 23.88,115.5 26.5,118.12 36.5,118.12 37.76,119.38 J1.4 43.24,119.38 44.5,118.12
L5
  Top 0.406: J6.5 46.34,116.84 47.62,118.12 59.12,118.12 61.62,115.62 84.88,115.62 86.25,117 J2.5 88.11,116.99 89.38,118.25 96,118.25 97.25,117 98.33,117 J7.5 99.1,116.97 100.38,118.25 109.25,118.25 111.75,115.75 123.12,115.75 123.25,115.62 127.62,115.62 129.12,117.12 138.57,117.12 J3.5 139.28,117.28 140.5,118.5 148.88,118.5 150,117.38 151.01,117.38 J8.5 151.66,117.28 152.88,118.5 166.75,118.5 169.12,116.12 192.5,116.12 193.62,117.24 J4.5 197.87,117.24 199.12,118.5 206.12,118.5 207.25,117.38 208.14,117.38 J9.5 208.53,117.28 209.75,118.5 249.12,118.5 250.5,117.12 252.32,117.12 J5.5 252.97,117.09 254.12,118.25 262.38,118.25 263.62,117 264.38,117 J10.5
  Top 0.506: X1.13 18.02,98.4 24.62,105 24.62,114.38 27.12,116.88 35.72,116.88 J1.5 36.34,116.84 37.62,118.12 43.12,118.12 44.38,116.88 45.88,116.88 J6.5
L6
  Top 0.406: J1.6 43.16,116.84 44.38,115.62 46.5,115.62 47.72,116.84 J6.6 57.91,116.84 61.62,113.12 83.5,113.12 86.12,115.75 88.38,115.75 89.61,116.99 J2.6 96.01,116.99 97.25,115.75 99,115.75 100.22,116.97 J7.6 109.03,116.97 112.88,113.12 127.75,113.12 130.62,116 139.36,116 140.65,117.28 J3.6 148.84,117.28 150.12,116 151.62,116 152.88,117.25 153.61,117.25 J8.6 165.72,117.28 169.5,113.5 191.25,113.5 193.62,115.88 197.87,115.88 199.24,117.24 J4.6 206.01,117.24 207.25,116 208.61,116 209.9,117.28 J9.6 221.59,117.28 223,115.88 250.88,115.88 251,115.75 252.75,115.75 254,117 254.8,117 J5.6 262.15,117.09 263.5,115.75 264.88,115.75 266.25,117.12 266.99,117.12 J10.6
  Top 0.506: X1.32 18,97 25.62,104.62 25.62,114 27.25,115.62 36.75,115.62 37.97,116.84 J1.6
L7
  Top 0.406: 37.88,115.5 36.67,114.3 J1.7 | J6.7 46.67,114.3 48,115.62 56.38,115.62 61.5,110.5 82.38,110.5 86.38,114.5 87.62,114.5 J2.7 88.58,114.45 89.88,115.75 96.12,115.75 97.5,114.38 98.3,114.38 J7.7 99.31,114.44 100.62,115.75 108,115.75 113.12,110.62 123.75,110.62 123.88,110.5 127.38,110.5 131.62,114.75 J3.7 139.25,114.75 140.62,116.12 148.75,116.12 150.12,114.75 J8.7 151.62,114.75 152.88,116 164.38,116 169.25,111.12 180.25,111.12 180.5,110.88 189.75,110.88 193.57,114.7 J4.7 198.07,114.7 199.38,116 206.12,116 207.38,114.75 J9.7 208.62,114.75 209.88,116 220.88,116 223.38,113.5 234,113.5 234.25,113.25 246,113.25 247.38,114.62 252.28,114.62 J5.7 253.06,114.56 254.38,115.88 262,115.88 263.25,114.62 264.41,114.62 J10.7
  Top 0.506: X1.14 18.26,95.63 26.38,103.75 26.38,112.12 28.62,114.38 35.67,114.38 J1.7 | 37.88,115.5 43.25,115.5 44.5,114.25 45.86,114.25 J6.7
L8
  Top 0.406: 29.88,113 36.5,113 37.8,114.3 J1.8 43.33,114.3 44.62,113 46.5,113 47.8,114.3 J6.8 55.45,114.3 61.88,107.88 80.88,107.88 86.12,113.12 88.51,113.12 89.83,114.45 J2.8 95.92,114.45 97.25,113.12 99.08,113.12 100.39,114.44 J7.8 106.56,114.44 113,108 127.25,108 132.75,113.5 139.12,113.5 140.25,114.62 141.15,114.62 J3.8 148.88,114.75 150.12,113.5 151.62,113.5 152.75,114.62 153.53,114.62 J8.8 162.88,114.75 169.12,108.5 180.25,108.5 180.5,108.25 188.38,108.25 193.5,113.38 198.12,113.38 199.45,114.7 J4.8 206.18,114.7 207.5,113.38 208.75,113.38 210.12,114.75 J9.8 220.38,114.75 222.25,112.87 222.25,112.25 223.62,110.88 234,110.88 234.12,110.75 245,110.75 247.5,113.25 252.97,113.25 254.27,114.56 J5.8 261.82,114.56 263.12,113.25 265.12,113.25 266.25,114.38 266.84,114.38 J10.8
  Top 0.506: X1.33 18.26,94.26 27.25,103.25 27.25,110.38 29.88,113
L9
  Top 0.406: J1.9 36.26,111.76 37.5,113 43.38,113 44.62,111.75 J6.9 46.26,111.76 47.5,113 54,113 61.62,105.38 79.88,105.38 86.38,111.88 87.64,111.88 J2.9 88.28,111.91 89.5,113.12 96.12,113.12 97.38,111.88 98.33,111.88 J7.9 99.02,111.89 100.38,113.25 105.5,113.25 113.25,105.5 123.75,105.5 123.88,105.38 127.38,105.38 134.12,112.12 138,112.12 138.25,112.38 138.56,112.38 J3.9 139.08,112.2 140.38,113.5 149,113.5 150.25,112.25 151.06,112.25 J8.9 151.71,112.2 153,113.5 161.88,113.5 169.38,106 180.62,106 180.88,105.75 187.5,105.75 193.88,112.12 197.53,112.12 J4.9 198.16,112.16 199.38,113.38 206.38,113.38 207.5,112.25 208.19,112.25 J9.9 208.83,112.2 210,113.38 220.25,113.38 221.38,112.25 221.38,110.38 223.38,108.38 234.12,108.38 234.25,108.25 243.75,108.25 247.5,112 252.34,112 J5.9 253.01,112.02 254.25,113.25 262,113.25 263.25,112 264.46,112 J10.9
  Top 0.506: X1.15 18.24,92.86 28.12,102.75 28.12,109.88 30.12,111.88 35.63,111.88 J1.9
L10
  Top 0.406: 36.25,110.5 37.51,111.76 J1.10 43.62,111.76 44.88,110.5 46.5,110.5 47.76,111.76 J6.10 52.74,111.76 61.5,102.88 78.62,102.88 86.38,110.62 88.12,110.62 89.38,111.88 89.62,111.88 89.75,111.75 90.05,111.75 J2.10 96.34,111.91 97.62,110.62 98.75,110.62 99.88,111.75 100.75,111.75 J7.10 100.92,111.88 103.75,111.88 112.5,103.12 112.5,103 112.62,102.88 128.5,102.88 136.5,110.88 139.5,110.88 140.75,112.12 141.19,112.12 J3.10 149.04,112.2 150.38,110.88 151.5,110.88 152.75,112.12 153.56,112.12 J8.10 153.69,112.25 160.62,112.25 169.5,103.38 180.62,103.38 180.75,103.25 186.12,103.25 193.75,110.88 198,110.88 199.28,112.16 J4.10 206.09,112.16 207.38,110.88 208.88,110.88 210.12,112.12 210.69,112.12 J9.10 220.04,112.2 220.62,111.62 220.62,108.5 223.25,105.88 233.75,105.88 234,105.62 242.88,105.62 248,110.75 253.13,110.75 254.4,112.02 J5.10 261.86,112.02 263.12,110.75 265.25,110.75 266.38,111.88 266.88,111.88 J10.10
  Top 0.506: X1.34 18.24,91.49 29,102.25 29,109.38 30.12,110.5 36.25,110.5
L11
  Top 0.406: J1.11 36.34,109.22 37.5,110.38 43.88,110.38 45,109.25 45.88,109.25 J6.11 46.47,109.22 47.75,110.5 52.38,110.5 61,101.88 78.88,101.88 86.38,109.38 J2.11 88,109.37 89.12,110.5 96.25,110.5 97.25,109.5 98.21,109.5 J7.11 98.86,109.36 100.12,110.62 102.62,110.62 112.88,100.38 128.25,100.38 137.5,109.62 138.69,109.62 J3.11 139.41,109.67 140.62,110.88 149.12,110.88 150.38,109.62 151.06,109.62 J8.11 151.54,109.67 152.88,111 159.38,111 169.5,100.88 180.75,100.88 180.88,100.75 185,100.75 193.88,109.62 J4.11 198.25,109.62 199.5,110.88 205.62,110.88 206.88,109.62 208.19,109.62 J9.11 208.91,109.67 210.12,110.88 219,110.88 219.88,110 219.88,106.75 223.38,103.25 234.25,103.25 234.38,103.12 241.75,103.12 248.12,109.5 252.33,109.5 J5.11 252.97,109.47 254.25,110.75 261.88,110.75 263.25,109.38 264.38,109.38 J10.11
  Top 0.506: X1.16 18.37,90.12 29.88,101.62 29.88,108.62 30.5,109.25 35.72,109.25 J1.11
L12
  Top 0.406: 31.5,108 36.25,108 37.5,109.25 38.26,109.25 J1.12 43.91,109.22 45.12,108 46.38,108 47.59,109.22 J6.12 52.16,109.22 60.25,101.12 79.38,101.12 86.38,108.12 88.5,108.12 89.75,109.37 J2.12 95.75,109.37 97.12,108 98.79,108 100.14,109.36 J7.12 102.27,109.36 111.88,99.75 111.88,98.5 112.5,97.88 127.38,97.88 137.62,108.25 139.35,108.25 140.77,109.67 J3.12 148.84,109.67 150.12,108.38 151.75,108.38 153,109.62 153.6,109.62 J8.12 158.21,109.67 169.5,98.38 180.38,98.38 180.5,98.25 185.5,98.25 195.5,108.25 198,108.25 199.25,109.5 199.99,109.5 J4.12 205.63,109.62 206.88,108.38 208.6,108.38 209.9,109.67 J9.12 218.21,109.67 219.12,108.75 219.12,104.88 223.25,100.75 234.12,100.75 234.38,100.5 240.62,100.5 248.38,108.25 253.04,108.25 254.27,109.47 J5.12 261.65,109.47 263,108.12 265,108.12 266.25,109.38 266.92,109.38 J10.12
  Top 0.506: X1.35 18.22,88.72 30.62,101.12 30.62,107.12 31.5,108
L13
  Top 0.406: J1.13 36.3,106.68 37.62,108 43.75,108 45,106.75 45.84,106.75 J6.13 46.3,106.68 47.5,107.88 52.38,107.88 59.88,100.38 79.75,100.38 86.25,106.88 87.62,106.88 J2.13 88.58,106.83 89.75,108 95.75,108 96.94,106.81 J7.13 98.69,106.81 99.88,108 101.75,108 102.12,107.62 102.12,107.5 104.75,104.88 104.75,104.38 110.88,98.25 111,98.25 112.25,97 127.5,97 132.12,101.62 132.12,101.75 137.5,107.12 J3.13 139.38,107.12 140.62,108.38 148.88,108.38 150.12,107.12 J8.13 151.75,107.12 153,108.38 156.62,108.38 169.25,95.75 180.88,95.75 181,95.62 184.75,95.62 196,106.88 197.37,106.88 J4.13 198.21,107.08 199.5,108.38 205.62,108.38 206.88,107.12 J9.13 208.75,107.12 210,108.38 217.75,108.38 218.38,107.75 218.38,103.12 223.38,98.12 239.38,98.12 248.25,107 252.29,107 J5.13 253.06,106.94 254.25,108.12 261.88,108.12 263.12,106.88 264.42,106.88 J10.13
  Top 0.506: X1.17 18.23,87.35 32.75,101.88 32.75,105.5 34,106.75 35.68,106.75 J1.13
L14
  Top 0.406: 34.88,105.5 36.38,105.5 37.55,106.68 J1.14 43.82,106.68 45.12,105.38 46.38,105.38 47.68,106.68 J6.14 52.57,106.68 59.62,99.62 80,99.62 86,105.62 88.5,105.62 89.7,106.83 J2.14 95.8,106.83 97,105.62 99.08,105.62 100.27,106.81 J7.14 101.5,106.81 102.56,105.75 102.62,105.75 103.62,104.75 103.62,104.25 111.62,96.25 127.75,96.25 137.25,105.75 139.27,105.75 140.65,107.12 J3.14 148.62,107.12 149.75,106 149.88,106 150,105.88 151.75,105.88 152.88,107 153.52,107 J8.14 155.25,107.12 169.88,92.62 184.5,92.62 188.06,96.06 188,96.12 188,97.62 196.12,105.75 198.16,105.75 199.49,107.08 J4.14 205.54,107.08 206.75,105.88 209.02,105.88 210.27,107.12 J9.14 217,107.12 217.75,106.38 217.75,101.25 223.38,95.62 234.62,95.62 234.75,95.5 238,95.5 248.25,105.75 253.34,105.75 254.52,106.94 J5.14 261.69,106.94 262.88,105.75 265.25,105.75 266.25,106.75 266.83,106.75 J10.14
  Top 0.506: X1.36 18.1,85.98 34.38,102.25 34.38,105 34.88,105.5
L15
  Top 0.406: J1.15 36.27,104.14 37.5,105.38 44,105.38 45.12,104.25 45.8,104.25 J6.15 46.52,104.14 47.75,105.38 52.75,105.38 59,99.12 59,99 59.12,98.88 80.62,98.88 86,104.25 87.63,104.25 J2.15 88.29,104.29 89.5,105.5 95.88,105.5 97.12,104.25 98.33,104.25 J7.15 98.9,104.28 100.25,105.62 101.5,105.62 102.12,105 102.12,104.75 111.38,95.5 128.25,95.5 137.38,104.62 138.69,104.62 J3.15 139.21,104.58 140.38,105.75 148.75,105.75 149.88,104.62 151.06,104.62 J8.15 151.71,104.58 153,105.88 155,105.88 169,91.88 185,91.88 188.88,95.75 188.88,97.38 196.12,104.62 197.49,104.62 J4.15 198.29,104.54 199.5,105.75 205.62,105.75 206.75,104.62 208.19,104.62 J9.15 208.96,104.58 210.12,105.75 216.5,105.75 217,105.25 217,99.38 223.38,93 234,93 234.12,92.88 238,92.88 239,93.88 239,95 248.5,104.5 252.25,104.5 J5.15 253.02,104.39 254.38,105.75 261.62,105.75 263,104.38 264.46,104.38 J10.15
  Top 0.506: X1.18 18.33,84.58 35.88,102.12 35.88,104.02 J1.15 35.73,104.12
L16
  Top 0.406: J1.16 43.73,104.14 45,102.88 47.19,102.88 J6.16 52.61,104.14 58.62,98.12 81.12,98.12 86,103 88.25,103 89.54,104.29 J2.16 95.71,104.29 97,103 98.87,103 100.14,104.28 J7.16 101.5,104.28 102,103.78 102,103.75 111,94.75 128.88,94.75 137.5,103.38 139.56,103.38 140.77,104.58 J3.16 148.16,104.58 149.5,103.25 151.5,103.25 152.75,104.5 153.56,104.5 J8.16 155.16,104.58 168.62,91.12 185.5,91.12 190,95.62 190,97.25 196,103.25 198.19,103.25 199.49,104.54 J4.16 205.46,104.54 206.75,103.25 208.75,103.25 210,104.5 210.69,104.5 J9.16 215.79,104.58 216.25,104.12 216.25,97.88 223.5,90.62 234.25,90.62 234.38,90.5 238.62,90.5 240.38,92.25 240.38,94.62 248.88,103.12 253.25,103.12 254.52,104.39 J5.16 261.86,104.39 263.12,103.12 265.12,103.12 266.38,104.38 267,104.38 J10.16
  Top 0.506: X1.37 18.34,83.21 38.25,103.12 38.25,104.1 J1.16
L17
  Top 0.406: J2.17 88.25,101.75 89.5,103 95.62,103 96.88,101.75 98.34,101.75 J7.17 98.86,101.73 100.12,103 101.5,103 102.25,102.25 102.38,102.25 110.62,94 129.25,94 137.25,102 138.69,102 J3.17 139.42,102.05 140.62,103.25 148.5,103.25 149.62,102.12 151.03,102.12 J8.17 151.29,102.05 152.5,103.25 155.25,103.25 168.12,90.38 185.75,90.38 190.75,95.38 190.75,96.75 196,102 J4.17 198.25,102 199.5,103.25 205.5,103.25 206.62,102.12 208.15,102.12 J9.17 208.79,102.05 210,103.25 214.88,103.25 215.5,102.62 215.5,97.5 223.12,89.88 234,89.88 234.25,89.62 239,89.62 241.12,91.75 241.12,94 249.12,102 252.21,102 J5.17 253.1,101.86 254.38,103.12 262,103.12 263.25,101.88 264.46,101.88 J10.17
  Top 0.506: J2.17 87.42,101.5 86,101.5 76.75,92.25 76.5,92.25 74.12,89.88 51.12,89.88 24.88,63.62 13.12,63.62 10.25,60.75 10.25,34.62 12.08,32.79 X2.11
L18
  Top 0.406: 88.25,100.5 89.5,101.75 J2.18 95.38,101.75 96.62,100.5 99.16,100.5 100.39,101.73 J7.18 100.91,101.75 101.62,101.75 110.12,93.25 129.5,93.25 137,100.75 139.38,100.75 140.67,102.05 J3.18 148.08,102.05 149.38,100.75 151.5,100.75 152.75,102 153.6,102 J8.18 155.33,102.05 167.75,89.62 186,89.62 191.5,95.12 191.5,96.25 196,100.75 198.24,100.75 199.49,102 J4.18 205.25,102 206.5,100.75 208.72,100.75 210.02,102.05 J9.18 214.21,102.05 214.75,101.5 214.75,97.25 222.88,89.12 233.62,89.12 234,88.75 240.38,88.75 242,90.38 242,93.75 248.88,100.62 253,100.62 254.12,101.75 254.79,101.75 J5.18 262.02,101.86 263.25,100.62 265,100.62 266.25,101.88 267,101.88 J10.18
  Top 0.506: 88.25,100.5 86.38,100.5 74.88,89 74.62,89 74.12,88.5 74,88.5 73.88,88.38 51.75,88.38 25.88,62.5 13.5,62.5 11.5,60.5 11.5,35.12 12.5,34.12 15,34.12 15.5,33.62 15.5,32.88 16.85,31.52 X2.30
L19
  Top 0.406: J2.19 88.21,99.21 89.5,100.5 95,100.5 96.31,99.19 J7.19 98.94,99.19 100.12,100.38 101.88,100.38 105.62,96.62 105.75,96.62 109.75,92.62 109.75,89.5 112,87.25 127,87.25 129.12,89.38 129.12,91.75 136.88,99.5 J3.19 139.25,99.5 140.5,100.75 148.12,100.75 149.38,99.5 J8.19 151.5,99.5 152.88,100.88 155.38,100.88 167.38,88.88 186.25,88.88 192.25,94.88 192.25,96 195.75,99.5 197.53,99.5 J4.19 198.21,99.46 199.5,100.75 205.5,100.75 206.75,99.5 J9.19 208.63,99.5 210,100.88 213.62,100.88 214,100.5 214,96.88 222.5,88.38 233.5,88.38 233.88,88 241.5,88 242.75,89.25 242.75,93.25 248.88,99.38 252.29,99.38 J5.19 252.94,99.31 254.25,100.62 262,100.62 263.25,99.38 264.42,99.38 J10.19
  Top 0.506: 87.58,99.12 J2.19 87.21,99.21 64.62,76.62 64.62,76.38 18.25,30 14.06,30 X2.12
L20
  Top 0.406: 90.12,99.12 J2.20 90.3,99.12 95.25,99.12 96.38,98 99.7,98 J7.20 100.97,99.12 102,99.12 108.88,92.25 108.88,89.25 111.62,86.5 127.5,86.5 130.12,89.12 130.12,91.75 136.62,98.25 139.38,98.25 140.63,99.5 J3.20 148.25,99.5 149.5,98.25 151.5,98.25 152.75,99.5 J8.20 155.75,99.5 167.12,88.12 186.5,88.12 193.12,94.75 193.12,95.62 195.75,98.25 198.4,98.25 199.61,99.46 J4.20 205.66,99.46 206.88,98.25 208.75,98.25 210,99.5 J9.20 212.62,99.5 213,99.12 213,96.88 222.88,87 241.75,87 243.62,88.88 243.62,93 248.62,98 252.88,98 254.19,99.31 J5.20 262.06,99.31 263.38,98 265,98 266.25,99.25 266.95,99.25 J10.20
  Top 0.506: X2.31 17.13,28.38 19.38,28.38 90.12,99.12
L21
  Top 0.406: J3.21 139.34,96.97 140.62,98.25 148.38,98.25 149.62,97 151.07,97 J8.21 151.72,96.97 153,98.25 155.88,98.25 166.88,87.25 187,87.25 194.12,94.38 194.12,95.12 195.88,96.88 197.53,96.88 J4.21 198.29,96.92 199.5,98.12 205.88,98.12 207,97 208.19,97 J9.21 208.84,96.97 210.12,98.25 212.12,98.25 212.25,98.12 212.25,96.75 222.62,86.38 242.25,86.38 244.5,88.62 244.5,92.75 248.5,96.75 252.33,96.75 J5.21 252.9,96.78 254.12,98 262,98 263.25,96.75 264.45,96.75 J10.21
  Top 0.506: X2.13 14.04,27.25 20,27.25 63.12,70.38 124,70.38 131,77.38 131,91.38 136.59,96.97 J3.21
L22
  Top 0.406: 139.31,95.62 140.65,96.97 J3.22 148.16,96.97 149.38,95.75 151.62,95.75 152.75,96.88 153.56,96.88 J8.22 156.03,96.97 166.5,86.5 187.38,86.5 194.88,94 194.88,94.62 195.88,95.62 198.31,95.62 199.61,96.92 J4.22 205.83,96.92 207.12,95.62 208.93,95.62 210.27,96.97 J9.22 211.03,96.97 222.25,85.75 242.62,85.75 245.38,88.5 245.38,92.5 248.5,95.62 253.25,95.62 254.4,96.78 J5.22 262.1,96.78 263.38,95.5 265.12,95.5 266.38,96.75 267,96.75 J10.22
  Top 0.506: X2.32 20.88,25.88 63.75,68.75 124,68.75 132,76.75 132,90.88 136.62,95.5 136.75,95.5 136.88,95.62 139.31,95.62
L23
  Top 0.406: J3.23 139.3,94.42 140.62,95.75 147.88,95.75 149.25,94.38 151.06,94.38 J8.23 151.68,94.42 153,95.75 156.12,95.75 166.12,85.75 187.88,85.75 196.62,94.5 197.45,94.5 J4.23 198.25,94.38 199.5,95.62 205.12,95.62 206.38,94.38 208.18,94.38 J9.23 208.8,94.42 210.12,95.75 211.25,95.75 216.88,90.12 216.88,83.5 220.75,79.62 239.38,79.62 246,86.25 246,92 248.38,94.38 252.22,94.38 J5.23 253.24,94.23 254.5,95.5 261.88,95.5 263.12,94.25 264.46,94.25 J10.23
  Top 0.506: X2.14 21.26,24.51 64,67.25 124.38,67.25 133.25,76.12 133.25,90 137.62,94.38 138.68,94.38 J3.23
L24
  Top 0.406: J3.24 147.57,94.42 148.88,93.12 151.5,93.12 152.75,94.38 153.59,94.38 J8.24 156.32,94.42 165.75,85 188.38,85 196.5,93.12 198.23,93.12 199.49,94.38 J4.24 204.87,94.38 206.12,93.12 208.59,93.12 209.9,94.42 J9.24 211.57,94.42 216,90 216,83 220,79 239.88,79 246.75,85.88 246.75,91.75 248,93 253.03,93 254.27,94.23 J5.24 261.76,94.23 263,93 265.25,93 266.5,94.25 267,94.25 J10.24
  Top 0.506: X2.33 22.26,23.14 64.38,65.25 124.38,65.25 134.62,75.5 134.62,89.5 137.88,92.75 139.59,92.75 J3.24
L25
  Top 0.406: 191.75,79 191.75,87.12 196.38,91.75 | J4.25 198.09,91.84 199.38,93.12 205,93.12 206.25,91.88 208.22,91.88 J9.25 208.63,91.89 210,93.25 211.62,93.25 215.12,89.75 215.12,82.75 219.75,78.12 240.12,78.12 247.5,85.5 247.5,90.88 248.25,91.62 252.28,91.62 J5.25 | 252.3,91.75 J5.25 | J5.25 253.07,91.69 254.38,93 261.75,93 263.12,91.62 264.41,91.62 J10.25
  Top 0.506: X2.15 22.62,21.74 25.62,24.75 25.75,24.75 64.12,63.12 175.88,63.12 191.75,79 | 196.38,91.75 197.48,91.75 J4.25
L26
  Top 0.406: 199.36,91.61 199.59,91.84 J4.26 204.91,91.84 206.38,90.38 209.26,90.38 J9.26 214.38,88.28 214.38,82.5 219.5,77.38 240.62,77.38 248.25,85 248.25,89.25 249.38,90.38 252.95,90.38 254.27,91.69 J5.26 261.81,91.69 263.12,90.38 265,90.38 266.25,91.62 266.95,91.62 J10.26
  Top 0.506: 199.36,91.61 197.5,89.75 195.75,89.75 193.12,87.12 193.12,78.5 176.25,61.62 65,61.62 23.75,20.38 X2.34
L27
  Top 0.406: X2.16 24.62,19 44.75,39.12 44.75,39.25 65.12,59.62 177.12,59.62 | J10.27 264.45,89.12 263.25,89.12 262,90.38 254.25,90.38 253.03,89.16 J5.27 252.32,89.12 250.62,89.12 249.62,88.12 249.62,85.38
  Top 0.506: 249.62,85.38 249,84.75 249,84.38 240.88,76.25 193.75,76.25 177.12,59.62
L28
  Top 0.406: 250.75,87.88 253.12,87.88 254.41,89.16 J5.28 261.85,89.16 263.12,87.88 265.38,87.88 266.5,89 266.87,89 J10.28 | 177.69,58.69 177.56,58.56 177.5,58.5
  Top 0.506: 177.5,58.5 65.88,58.5 24.88,17.5 16.95,17.5 X2.35 | 250.75,87.88 250.75,85.25 250.12,84.62 250.12,83.88 241.38,75.12 194.12,75.12 177.56,58.56 | 177.75,58.75 177.69,58.69
L29
  Top 0.406: 25.25,16.12 14.11,16.12 X2.17 | J5.29 252.99,86.61 254.25,87.88 261.75,87.88 263,86.62 264.47,86.62 J10.29
  Top 0.506: 25.25,16.12 66.62,57.5 178.12,57.5 178.25,57.62 178.5,57.62 194.88,74 241.5,74 252.35,84.86 J5.29
L30
  Top 0.406: J5.30 261.38,86.61 263,85 265.4,85 J10.30
  Top 0.506: J5.30 254.9,86.02 242,73.12 195.75,73.12 178.75,56.12 67.38,56.12 26.5,15.25 26.5,15.12 26.12,14.75 16.96,14.75 X2.36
